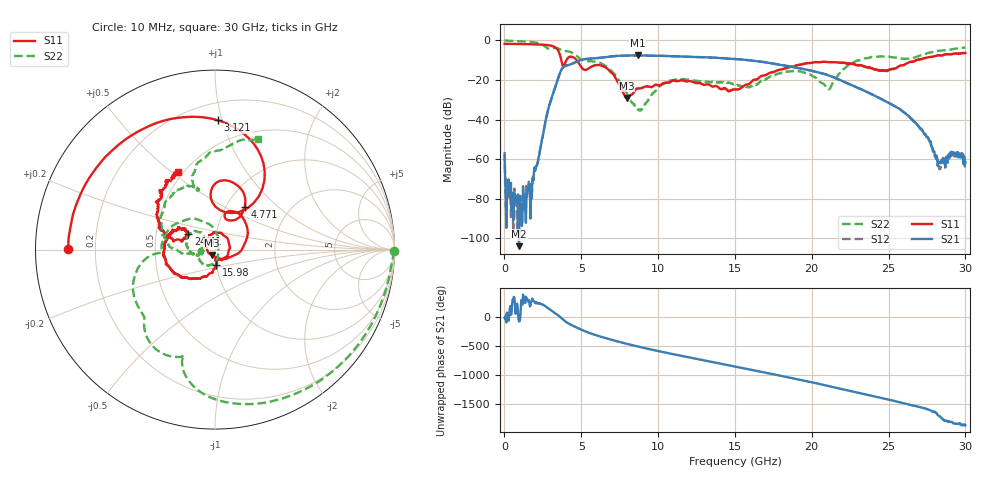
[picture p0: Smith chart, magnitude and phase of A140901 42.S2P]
!  2-Port S-parameters saved by WinCal
! VAR MeasName=S-Parameters (CALIBRATED_DATA) read from VNA (N5244A)
! VAR MeasDate=11/3/2014 9:33:53 AM
! VAR NAME=A140901 42
! VAR FILENAME=A140901 42.S2P
! VAR DATE=11/3/2014 9:33:53 AM
! VAR PHYS_PORTS=1,2
# Hz S RI R 50
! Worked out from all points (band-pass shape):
!   801 points, 10 MHz to 30 GHz, reference 50 ohm
!   highest |S21| = -7.55 dB at 8.67 GHz (marker M1); lowest = -103.9 dB at 947.2 MHz (marker M2)
!   |S21| within 3 dB of the highest: 4.745 GHz to 16.46 GHz (11.72 GHz wide, 111 % of centre)
!   lowest |S11| = -29.0 dB at 7.957 GHz (marker M3), VSWR 1.07, Z = 48.1 - j2.93 ohm
!   |S11| at or under -10 dB: 3.699 GHz to 4.033 GHz (334.7 MHz wide, 8.66 % of centre); 4.702 GHz to 26.77 GHz (22.07 GHz wide, 140 % of centre); 26.78044 GHz to 26.82275 GHz (42.31 MHz wide, 0.158 % of centre)
!   |S22| runs from -35.5 to 0.0 dB; largest |S21 - S12| = 0.0025
!   S11 on the Smith chart (normalised r, x): 10 MHz: 0.10, +0.00; 3.121 GHz: 0.32, +0.97; 4.771 GHz: 1.21, +0.64; 15.98 GHz: 1.00, -0.17; 24.41 GHz: 0.73, +0.14; 30 GHz: 0.47, +0.53
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1e7  -0.818 0.00226  0.00118 -0.000392  -0.000342 -0.00149  0.9968 -0.00783
1.974375e8  -0.8151 0.0647  5.82e-05 -0.000128  -0.000221 1.26e-05  0.9746 -0.1312
9.471875e8  -0.7525 0.3018  8.22e-07 -6.33e-06  -2.75e-06 -1.02e-05  0.7854 -0.5455
1.771912e9  -0.5911 0.5361  -5.29e-06 -0.000101  9.89e-05 -5.12e-05  0.3627 -0.8331
3.121462e9  0.0169 0.7204  5.45e-05 0.0406  0.000233 0.0407  -0.2087 -0.5985
3.796238e9  0.0955 0.2035  0.1434 -0.1464  0.1431 -0.1454  -0.3937 -0.3813
4.770912e9  0.1654 0.2396  -0.2894 0.0785  -0.2891 0.0781  -0.3828 -0.0482
5.033325e9  0.1178 0.1681  -0.223 0.2367  -0.2233 0.2362  -0.3243 -0.0217
6.495338e9  0.1807 0.1179  0.3742 -0.00728  0.3742 -0.00606  -0.1737 0.1618
7.95735e9  -0.018 -0.0304  -0.1161 -0.3981  -0.1154 -0.3985  0.0195 0.0433
8.669612e9  -0.0543 0.028  -0.3708 -0.1959  -0.3704 -0.1959  0.018 0.00196
1.001916e10  -0.0378 0.0629  -0.2551 0.3211  -0.2545 0.3207  0.00478 -0.0638
1.238088e10  0.0759 0.0383  0.3819 0.0111  0.3813 0.0116  -0.09 -0.0349
1.5005e10  0.0062 -0.0565  -0.2443 -0.2342  -0.2442 -0.2346  -0.0762 0.00398
1.597968e10  0.00524 -0.0834  -0.3112 0.0462  -0.3116 0.0456  -0.068 -0.00878
2.002832e10  -0.2567 -0.0954  0.1116 -0.1276  0.1123 -0.1281  -0.0813 0.0963
2.111546e10  -0.2801 0.00335  -0.0532 -0.119  -0.0531 -0.1187  -0.0558 0.0182
2.441436e10  -0.1477 0.0895  0.0231 0.0262  0.023 0.0265  -0.2247 0.3253
2.501416e10  -0.1626 0.0636  0.0258 0.00576  0.0258 0.00592  -0.1528 0.3563
2.722592e10  -0.3067 0.1507  -0.00317 -0.00418  -0.00308 -0.00412  -0.1271 0.4116
2.831306e10  -0.3256 0.2657  1.87e-05 0.000809  -0.000112 0.000543  -0.00628 0.5476
3e10  -0.2082 0.4327  0.000352 -0.000766  0.000261 -0.000852  0.2372 0.6176
